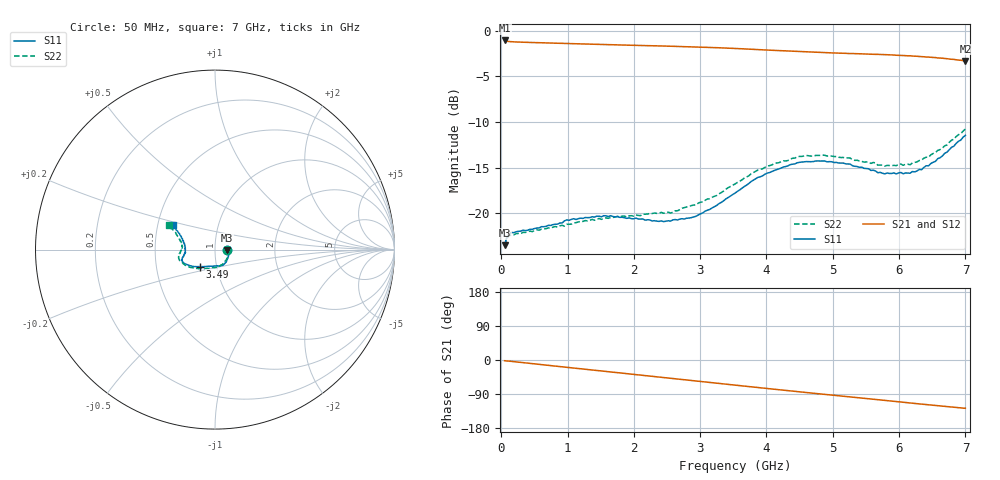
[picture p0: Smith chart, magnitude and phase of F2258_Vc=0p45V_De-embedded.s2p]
! Integrated Device Technology
! Corporate Headquarters
! 6024 Silver Creek Valley Road
! San Jose, CA 95138  USA
! Phone:  1-408-284-8200
! Toll Free:  1-800-223-1366
! Webpage:  http://www.idt.com/
! Timing and RF Division
! 515 Groton Road, Suite 102
! Westford, MA 01886-6024
! Device:  F2258
! Description: Voltage Variable RF Attenuator
! Frequency:  50.0 -  6000.00 MHz
! Package:  3x3 mm Thin QFN Plastic Package: 16 pin
! Ports:  2 RF, 2 DC
!  Pin  1  = NC
!  Pin  2  = NC
!  Pin  3  = RF2  = Port 2
!  Pin  4  = GND
!  Pin  5  = Vdd
!  Pin  6  = NC
!  Pin  7  = VCTRL
!  Pin  8  = NC
!  Pin  9  = GND
!  Pin 10  = RF1  = Port 1
!  Pin 11  = NC
!  Pin 12  = NC
!  Pin 13  = NC
!  Pin 14  = NC
!  Pin 15  = NC
!  Pin 16  = NC
! Vcntrl:  0.450 Volts
! Vdd:  +3.300 Volts
! Current:  1.096 mA
! Data:  The device was measured on a the F2258 evaluation board which has
!  individual transmission lines to the RF pins.  Data was collected
!  using a calibrated network analyzer.  The evaluation board was
!  de-embedded using a TRL calibration technique.
!  The reference plane is the edge of the package pin.
! Misc:  SN 10
!  Action Tracker AT0285
! Date Measured:  2014-12-10
! Date:  2016-01-13  MJV
! Note:
!  Integrated Device Technology supplies this data as a sample of measured
!  data at the package pin for this product.  Your particular data for this
!  product may vary.
!  Data was taken at 25 degrees C.
!  Integrated Device Technology reserves the right to change this data at anytime.
!Freq_(GHz)  S11M_(dB)  S11P_(deg)  S21M_(dB)  S21P_(deg)  S12M_(dB)  S12P_(deg)  S22M_(dB)  S22P_(deg)
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# GHz S dB R 50
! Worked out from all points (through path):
!   201 points, 50 MHz to 7 GHz, reference 50 ohm
!   highest |S21| = -1.05 dB at 50 MHz (marker M1); lowest = -3.3 dB at 7 GHz (marker M2)
!   group delay of S21, straight-line fit = 50.5 ps
!   lowest |S11| = -23.5 dB at 50 MHz (marker M3), VSWR 1.14, Z = 57.2 - j0.434 ohm
!   |S11| at or under -10 dB: start of sweep to end of sweep
!   |S22| runs from -23.6 to -10.8 dB; largest |S21 - S12| = 0.0004
!   S11 on the Smith chart (normalised r, x): 50 MHz: 1.14, -0.01; 3.49 GHz: 0.83, -0.16; 7 GHz: 0.60, +0.17
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0.05  -23.48 -3.2  -1.05 -2.0  -1.05 -2.0  -23.59 -3.1
0.08475  -22.55 -5.3  -1.14 -2.5  -1.13 -2.5  -22.69 -5.1
0.15425  -22.08 -8.2  -1.19 -3.7  -1.19 -3.7  -22.33 -8.9
0.71025  -21.30 -33.5  -1.33 -14.1  -1.33 -14.1  -21.59 -36.4
0.98825  -20.72 -46.5  -1.38 -19.4  -1.38 -19.4  -21.19 -51.7
1.2315  -20.55 -54.3  -1.43 -23.8  -1.43 -23.8  -20.88 -60.6
1.6485  -20.26 -65.6  -1.52 -31.4  -1.52 -31.4  -20.45 -73.7
2.37825  -20.87 -85.7  -1.65 -44.8  -1.65 -44.8  -19.97 -92.0
2.552  -20.84 -91.5  -1.68 -48.0  -1.68 -48.0  -19.95 -97.3
2.93425  -20.32 -108.2  -1.76 -55.1  -1.76 -55.1  -19.07 -110.8
3.49025  -17.93 -131.7  -1.92 -65.6  -1.91 -65.6  -16.92 -132.4
3.525  -17.78 -132.7  -1.93 -66.2  -1.92 -66.2  -16.78 -133.9
4.0115  -15.59 -147.5  -2.11 -75.3  -2.11 -75.3  -14.82 -149.6
4.46325  -14.45 -156.5  -2.27 -83.4  -2.27 -83.4  -13.81 -160.9
4.7065  -14.32 -159.8  -2.34 -87.7  -2.34 -87.7  -13.71 -165.2
5.2625  -14.60 -166.5  -2.49 -97.4  -2.49 -97.4  -13.94 -173.5
5.6795  -15.54 -173.0  -2.57 -104.6  -2.58 -104.6  -14.72 -179.1
5.85325  -15.63 -177.2  -2.63 -107.8  -2.63 -107.8  -14.75 176.3
6.166  -15.60 174.9  -2.74 -113.4  -2.74 -113.3  -14.67 170.2
6.33975  -15.21 168.3  -2.82 -116.5  -2.82 -116.5  -14.15 165.8
6.722  -13.29 155.8  -3.05 -123.1  -3.05 -123.1  -12.50 156.7
7  -11.45 149.9  -3.30 -127.4  -3.30 -127.4  -10.77 151.7
